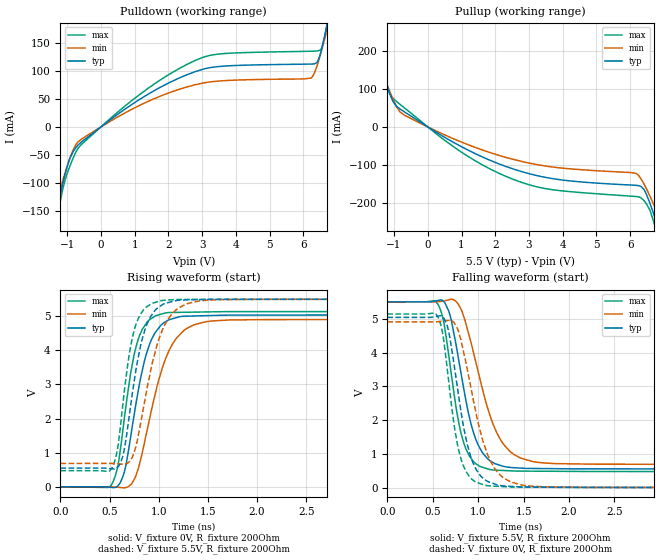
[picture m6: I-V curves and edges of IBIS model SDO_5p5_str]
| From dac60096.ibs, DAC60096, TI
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|   Model
[Model]   SDO_5p5_str
Model_type   Output
Polarity   Non-Inverting
Vmeas = 2.75
Vref = 0
Cref = 1pF
Rref = 100000
|   typ   min   max
C_comp   13.124pF   12.937pF   13.913pF
[Voltage Range]   5.5   5.499   5.501
[Temperature Range]   27   105   -40
[Pullup Reference]   5.5   5.499   5.501
[Pulldown Reference]   0   0   0
[Power Clamp Reference]   5.5   5.499   5.501
[GND Clamp Reference]   0   0   0
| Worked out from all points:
|   slope of the pulldown table from 0 to 0.825 V, typ, clamps not added: 22.7 ohm
|   slope of the pullup table from 0 to 0.825 V, typ, clamps not added: 18.9 ohm
|   falling waveform, V_fixture 5.5V, R_fixture 200Ohm: 20-80 % time 224ps typ, 305ps min, 180ps max; typ from 5.5 V to 0.548 V
|   rising waveform, V_fixture 0V, R_fixture 200Ohm: 20-80 % time 200ps typ, 264ps min, 163ps max; typ from 0 V to 5.04 V
|   rising waveform, V_fixture 5.5V, R_fixture 200Ohm: 20-80 % time 176ps typ, 227ps min, 144ps max; typ from 0.548 V to 5.5 V
|   falling waveform, V_fixture 0V, R_fixture 200Ohm: 20-80 % time 196ps typ, 256ps min, 161ps max; typ from 5.04 V to 0 V
[Pulldown]
|   Voltage   I(typ)   I(min)   I(max)
-5.5V     -1.396A    -1.141A    -1.674A
-1.887V   -311.7mA   -259.1mA   -367.9mA
-1.359V   -161.5mA   -142mA     -182.9mA
-946mV    -60.14mA   -60.38mA   -73.98mA
-583mV    -27.09mA   -21.96mA   -31.43mA
1.397V    58.22mA    45.43mA    68.71mA
3.014V    102.6mA    78mA       123.7mA
6.231V    112mA      87.08mA    134.8mA
6.396V    114.2mA    106.7mA    135.2mA
6.529V    135mA      133.3mA    138.6mA
6.726V    187.7mA    177.8mA    190.5mA
11V       1.533A     1.256A     1.891A
[Pullup]
|   Voltage   I(typ)   I(min)   I(max)
-5.5V     1.434A     1.169A     1.793A
-1.804V   284mA      251.8mA    328.7mA
-1.127V   87.72mA    93.02mA    87.3mA
-814mV    46.73mA    38.68mA    58.63mA
1.117V    -57.45mA   -44mA      -73.15mA
2.783V    -117.5mA   -90.75mA   -145.9mA
6.165V    -153.5mA   -121.9mA   -182.9mA
6.413V    -165mA     -150.5mA   -194.1mA
6.726V    -236.2mA   -209.7mA   -258mA
6.875V    -276.2mA   -240.7mA   -307.1mA
7.42V     -431.6mA   -361.7mA   -499.2mA
11V       -1.511A    -1.24A     -1.802A
[Ramp]
R_load = 200
|   typ   min   max
dV/dt_r   3.02435/1.99602e-10   2.94371/2.63124e-10   3.08421/1.6276e-10
dV/dt_f   2.97105/2.22989e-10   2.88812/3.03573e-10   3.01696/1.79212e-10
[Falling Waveform]
V_fixture = 5.5V
V_fixture_min = 5.499V
V_fixture_max = 5.501V
R_fixture = 200Ohm
C_fixture = 0F
|   Time   V(typ)   V(min)   V(max)
0s        5.5V       5.499V     5.501V
515ps     5.518V     5.499V     5.531V
632.2ps   5.477V     5.53V      4.729V
703.5ps   4.959V     5.58V      3.382V
831.7ps   3.074V     5.141V     1.414V
961.7ps   1.527V     3.854V     742.8mV
1.123ns   815.4mV    2.196V     545.2mV
1.355ns   603.7mV    1.066V     504.2mV
1.714ns   570.9mV    738.4mV    491.8mV
10ns      548.3mV    685.5mV    472.7mV
[Rising Waveform]
V_fixture = 0V
V_fixture_min = 0V
V_fixture_max = 0V
R_fixture = 200Ohm
C_fixture = 0F
|   Time   V(typ)   V(min)   V(max)
0s        -23.28nV   -37.81nV   -23.11nV
503.2ps   -13.34mV   1.248mV    3.17mV
600.3ps   82.67mV    -18.06mV   898.5mV
709.3ps   1.371V     50.42mV    3.238V
793.1ps   2.844V     543.7mV    4.34V
915.8ps   4.245V     2.115V     4.916V
1.068ns   4.837V     3.747V     5.096V
1.287ns   5.002V     4.646V     5.117V
1.714ns   5.034V     4.89V      5.135V
10ns      5.041V     4.906V     5.14V
[Rising Waveform]
V_fixture = 5.5V
V_fixture_min = 5.499V
V_fixture_max = 5.501V
R_fixture = 200Ohm
C_fixture = 0F
|   Time   V(typ)   V(min)   V(max)
0s        548.1mV    684.9mV    472.7mV
504ps     533.7mV    686.1mV    474.7mV
594.9ps   617.5mV    668.3mV    1.407V
652.4ps   1.139V     659.1mV    2.869V
755.7ps   3.199V     1.065V     4.643V
865.7ps   4.655V     2.647V     5.253V
1.016ns   5.296V     4.443V     5.452V
1.204ns   5.466V     5.247V     5.489V
1.6ns     5.493V     5.483V     5.496V
10ns      5.5V       5.499V     5.501V
[Falling Waveform]
|Gnd
V_fixture = 0V
V_fixture_min = 0V
V_fixture_max = 0V
R_fixture = 200Ohm
C_fixture = 0F
|   Time   V(typ)   V(min)   V(max)
0s        5.041V     4.906V     5.14V
533.3ps   5.066V     4.906V     5.145V
622.8ps   5.019V     4.935V     4.315V
687.3ps   4.454V     4.957V     2.876V
804.2ps   2.372V     4.431V     918.4mV
915.8ps   939.6mV    3.015V     295.2mV
1.068ns   256.1mV    1.255V     79.91mV
1.287ns   55.14mV    279.7mV    35.39mV
1.714ns   21.24mV    31.16mV    19.5mV
10ns      258.2uV    795.3uV    49.14uV
